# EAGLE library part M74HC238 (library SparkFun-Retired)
M74HC238 - CMOS 3 TO 8 LINE DECODER RETIRED: IC-09771
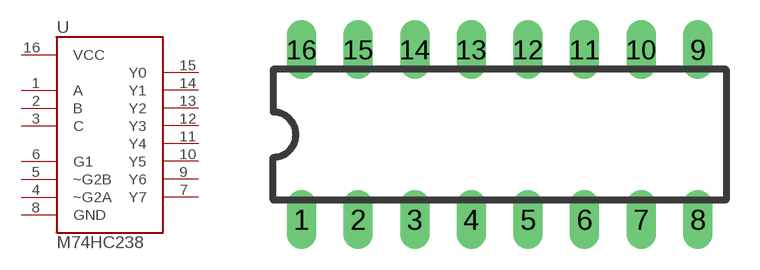
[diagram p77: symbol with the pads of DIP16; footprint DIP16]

Designator prefix -

## M74HC238  [DIP16]
1  A
2  B
3  C
4  ~G2A
5  ~G2B
6  G1
7  Y7
8  GND
9  Y6
10  Y5
11  Y4
12  Y3
13  Y2
14  Y1
15  Y0
16  VCC

## Footprint DIP16 (pad centres in mm)
Dual In Line Package
drill 0.813 long: 1 -8.89,-3.81; 2 -6.35,-3.81; 3 -3.81,-3.81; 4 -1.27,-3.81; 5 1.27,-3.81; 6 3.81,-3.81; 7 6.35,-3.81; 8 8.89,-3.81; 9 8.89,3.81; 10 6.35,3.81; 11 3.81,3.81; 12 1.27,3.81; 13 -1.27,3.81; 14 -3.81,3.81; 15 -6.35,3.81; 16 -8.89,3.81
